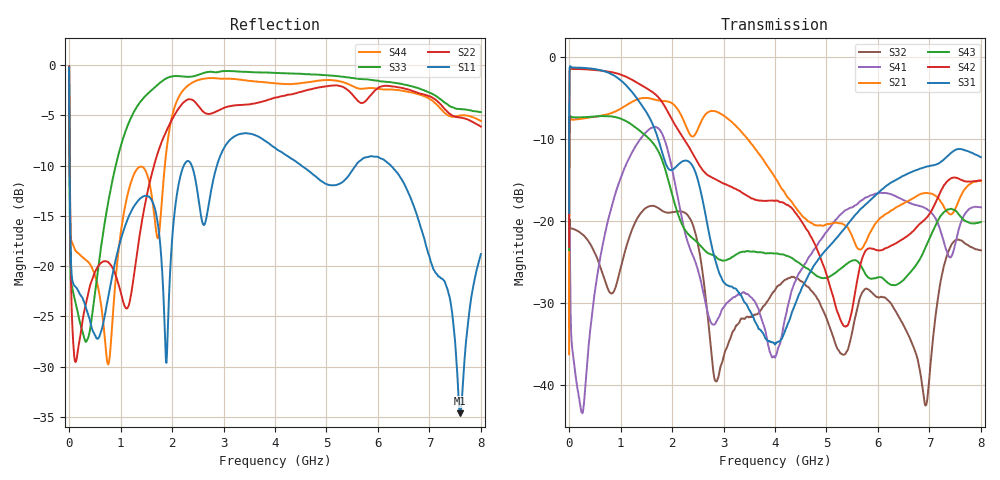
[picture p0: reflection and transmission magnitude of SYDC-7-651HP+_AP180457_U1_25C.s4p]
!Created: 06-20-2018 at 12:37:35
!Mini-Circuits
!S4P DATA File Format
!Type: Directional Coupler
!MODEL: SYDC-7-651HP+
!S/N: Unit 1
!TEST CONDITIONS: Z:50 OHM SYSTEM, INPUT POWER = 0dBm, TEMP:25°C
!REMARK: Full 2 port calibration using Ecal. Port  extension done.
!TESTED ON: NETWORK ANALYZER MODEL E5071C S/N 76113 CAL DUE DATE 05/10/19
# MHZ S DB R 50
!Frequency  S11 dB  S11 DEG  S12 dB  S12 DEG  S13 dB  S13 DEG  S14 dB  S14 DEG
!  S21 dB  S21 DEG  S22 dB  S22 DEG  S23 dB  S23 DEG  S24 dB  S24 DEG
!  S31 dB  S31 DEG  S32 dB  S32 DEG  S33 dB  S33 DEG  S34 dB  S34 DEG
!  S41 dB  S41 DEG  S42 dB  S42 DEG  S43 dB  S43 DEG  S44 dB  S44 DEG
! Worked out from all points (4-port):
!   1501 points, 300 kHz to 8 GHz, reference 50 ohm
!   strongest paths, dB at 300 kHz, 675 kHz, 500 MHz, 4.25 GHz, 8 GHz:
!     S31: -19.0, -12.3, -1.5, -32.5, -12.2
!     S42: -23.2, -16.3, -1.6, -18.1, -15.1
!     S43: -23.6, -16.9, -7.3, -24.3, -20.1
!     S21: -36.3, -28.7, -7.3, -17.2, -15.2
!     S41: -30.0, -23.4, -28.6, -30.4, -18.3
!     S32: -33.0, -26.3, -23.9, -27.0, -23.6
!   lowest |S11| = -34.6 dB at 7.59 GHz (marker M1), VSWR 1.04, Z = 50.5 - j1.79 ohm
!   |S11| at or under -10 dB: 9.473 MHz to 2.227 GHz (2.218 GHz wide, 198 % of centre); 4.516 GHz to 5.565 GHz (1.05 GHz wide, 20.8 % of centre); 6.254 GHz to end of sweep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
0.3  -0.21 173.1  -36.31 91.4  -18.99 79.9  -29.92 -101.6
     -36.26 91.1  -0.12 175.8  -32.96 -99.5  -23.01 82.4
     -19.02 80.0  -32.98 -99.6  -0.09 172.9  -23.52 -98.4
     -30.01 -101.8  -23.16 82.1  -23.55 -98.9  -0.17 175.2
1  -0.79 158.2  -24.62 94.0  -9.34 65.5  -20.48 -127.2
   -24.63 93.5  -0.43 165.5  -23.42 -120.5  -13.03 72.8
   -9.35 65.6  -23.41 -120.1  -0.83 157.6  -13.90 -116.2
   -20.54 -127.1  -13.09 73.1  -13.92 -116.2  -0.64 164.6
90  -21.86 6.2  -7.65 0.6  -1.29 -6.3  -37.00 122.4
    -7.66 0.6  -28.38 30.2  -21.05 168.2  -1.45 -4.5
    -1.31 -6.3  -21.00 168.2  -22.86 165.9  -7.37 167.8
    -37.14 121.5  -1.48 -4.5  -7.37 167.8  -18.07 163.8
1660  -14.14 -51.8  -5.20 -67.0  -8.71 -157.9  -8.50 42.9
      -5.22 -66.9  -9.78 -54.9  -18.13 61.8  -4.48 -135.0
      -8.76 -157.7  -18.20 62.4  -2.22 -131.9  -10.79 -95.6
      -8.55 42.7  -4.49 -135.1  -10.76 -96.0  -15.17 -110.8
3960  -8.10 -55.3  -14.25 128.0  -34.62 75.1  -37.42 31.8
      -14.29 127.1  -3.30 -150.0  -28.81 12.3  -17.50 80.9
      -34.82 65.0  -28.70 11.0  -0.75 132.5  -23.84 21.4
      -36.60 16.1  -17.51 80.2  -23.96 21.9  -1.78 174.6
7590  -34.64 -72.4  -16.98 -145.6  -11.28 110.4  -20.40 -143.5
      -17.23 -145.0  -5.20 56.1  -22.13 -13.7  -14.94 -163.6
      -11.24 109.8  -22.34 -14.3  -4.36 -3.7  -19.44 20.1
      -20.61 -142.8  -14.94 -164.6  -19.37 18.8  -5.02 37.5
8000  -18.80 -22.2  -14.88 178.2  -12.07 73.9  -18.03 165.8
      -15.16 177.7  -6.11 49.8  -23.44 -56.9  -15.18 151.0
      -12.24 71.8  -23.58 -56.1  -4.66 -9.7  -20.50 -5.4
      -18.35 164.0  -15.07 151.2  -20.14 -4.6  -5.55 27.9
